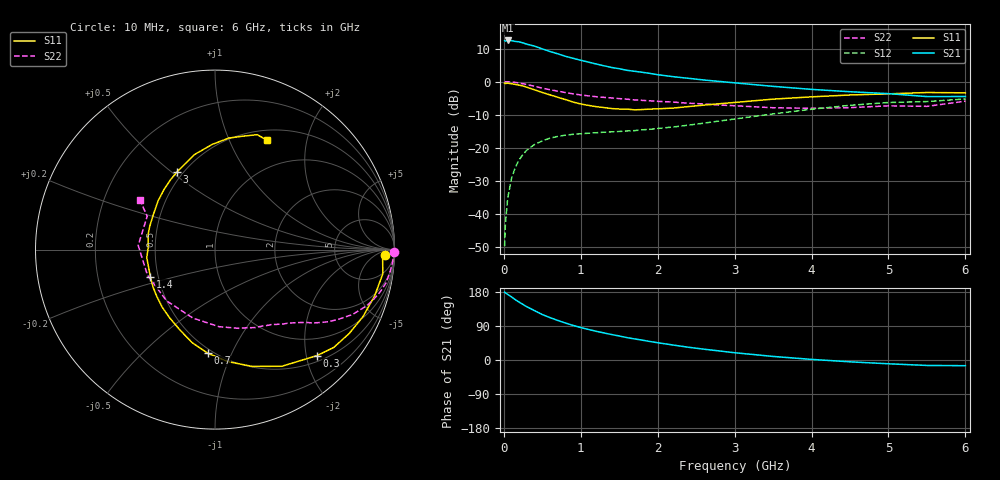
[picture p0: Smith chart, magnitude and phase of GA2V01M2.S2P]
! Infineon Technologies  Discrete & RF Semiconductors
! BF775
! Si NPN RF Bipolar Junction Transistor in SOT23
! VCE = 2 V  IC = 1.2 mA
! Common Emitter S-Parameters:  May  1996
# GHz  S  MA  R  50
!  f  S11  S21  S12  S22
! GHz  MAG  ANG  MAG  ANG  MAG  ANG  MAG  ANG
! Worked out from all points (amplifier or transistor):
!   36 points, 10 MHz to 6 GHz, reference 50 ohm
!   highest |S21| = 12.5 dB at 50 MHz (marker M1)
!   |S21| within 3 dB of that: start of sweep to 556.6 MHz
!   unconditionally stable (mu >= 1): 1.334 GHz to end of sweep
!   at 250 MHz: K = 0.22, MSG = 16.9 dB, |S12| = -22.1 dB
!   at 1.4 GHz: K = 1.04, MAG = 8.5 dB, |S12| = -15.3 dB
!   at 6 GHz: K = 1.05, MAG = -0.9 dB, |S12| = -5.3 dB
!   S11 on the Smith chart (normalised r, x): 10 MHz: 28, -15; 300 MHz: 0.61, -2.21; 700 MHz: 0.47, -0.81; 1.4 GHz: 0.45, -0.16; 3 GHz: 0.46, +0.52; 6 GHz: 0.62, +1.39
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0.01  0.9459 -1.7  4.165 179.0  0.0032 88.0  1 -0.7
0.02  0.9355 -3.2  4.095 177.2  0.0069 87.3  0.9893 -1.5
0.05  0.9447 -8.2  4.196 173.1  0.017 85.6  0.9927 -3.8
0.1  0.926 -16.2  4.163 166.5  0.0341 79.8  0.9825 -7.5
0.15  0.9052 -24.3  4.054 159.0  0.0505 75.2  0.9701 -11.1
0.2  0.8819 -32.0  4.002 152.6  0.0654 70.5  0.9497 -14.4
0.3  0.8196 -46.1  3.681 140.4  0.0915 62.5  0.9013 -20.3
0.4  0.7491 -60.2  3.442 130.1  0.1115 55.3  0.848 -25.2
0.5  0.6831 -72.3  3.127 119.9  0.1262 49.9  0.7943 -29.1
0.6  0.6284 -83.4  2.856 111.9  0.1387 45.1  0.7526 -32.2
0.7  0.5783 -94.1  2.635 104.5  0.1473 41.8  0.7154 -34.6
0.9  0.4893 -113.4  2.252 91.3  0.1586 37.0  0.6508 -38.6
1.1  0.4352 -132.6  1.971 80.7  0.1649 34.4  0.6065 -42.2
1.4  0.3901 -157.3  1.635 67.2  0.1726 32.6  0.5644 -47.2
1.7  0.3727 179.0  1.431 55.6  0.1804 34.3  0.5266 -52.3
2.2  0.3961 149.7  1.186 39.5  0.2048 37.3  0.4886 -62.8
3  0.4822 116.1  0.956 19.2  0.2704 39.2  0.4301 -87.0
3.5  0.5415 102.2  0.846 9.4  0.3235 36.4  0.401 -107.8
4.5  0.626 83.0  0.701 -4.8  0.4368 24.9  0.4023 -159.2
5  0.6511 76.1  0.656 -10.0  0.4812 17.3  0.4286 176.9
5.5  0.6822 69.8  0.592 -14.4  0.4978 8.9  0.4209 153.8
6  0.6746 64.5  0.593 -15.0  0.5448 4.4  0.5041 146.4
